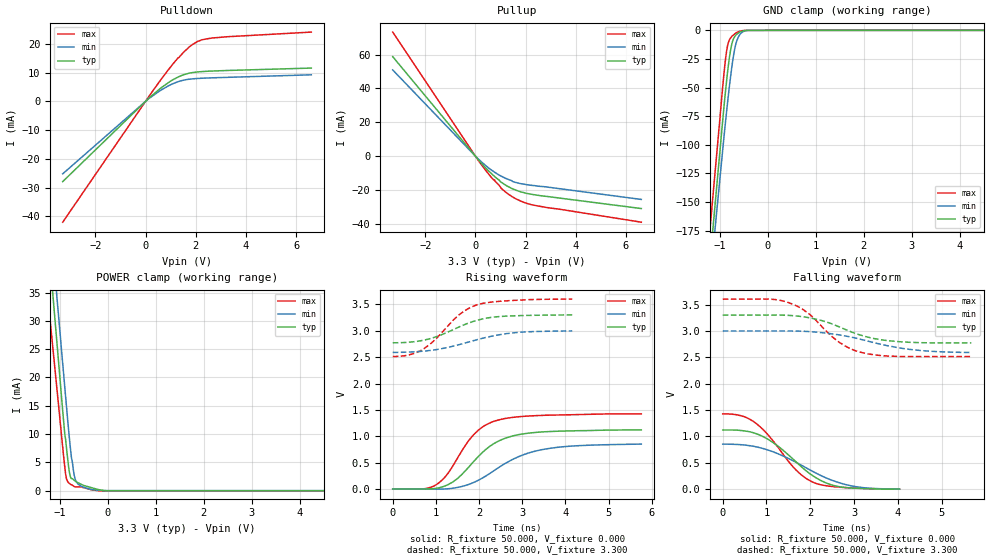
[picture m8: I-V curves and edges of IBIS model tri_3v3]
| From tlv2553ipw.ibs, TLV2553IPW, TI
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[Model]   tri_3v3
Model_type 3-state
Vref=0.000E+00
Rref=5.000E+06
Cref=3.000E-11
Vmeas=1.65E+00
C_comp  2.00000pF 2.00000pF 2.00000pF
[Voltage Range]   3.300E+00   3.000E+00   3.600E+00
[POWER Clamp Reference]   3.300E+00   3.000E+00   3.600E+00
[GND Clamp Reference]   0.000E+00   0.000E+00   0.000E+00
[Pullup Reference]   3.300E+00   3.000E+00   3.600E+00
[Pulldown Reference]   0.000E+00   0.000E+00   0.000E+00
[Temperature Range]   25   105   -40
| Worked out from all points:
|   slope of the pulldown table from 0 to 0.495 V, typ, clamps not added: 130 ohm
|   slope of the pullup table from 0 to 0.495 V, typ, clamps not added: 59.8 ohm
|   GND clamp passes 1 mA (typ) near -0.56 V on its own axis
|   POWER clamp passes 1 mA (typ) near -0.53 V on its own axis
|   rising waveform, R_fixture 50.000, V_fixture 0.000: 20-80 % time 888ps typ, 1.15ns min, 752ps max; typ from 0.001 V to 1.12 V
|   falling waveform, R_fixture 50.000, V_fixture 0.000: 20-80 % time 987ps typ, 1.26ns min, 867ps max; typ from 1.12 V to 0.001 V
|   rising waveform, R_fixture 50.000, V_fixture 3.300: 20-80 % time 969ps typ, 1.21ns min, 839ps max; typ from 2.77 V to 3.3 V
|   falling waveform, R_fixture 50.000, V_fixture 3.300: 20-80 % time 1.07ns typ, 1.37ns min, 895ps max; typ from 3.3 V to 2.77 V
[GND Clamp]
-3.3V     -1.173A    -1.124A    -1.155A
-1.02V    -115.5mA   -138.7mA   -86.59mA
-900mV    -60.5mA    -87.21mA   -31.75mA
-840mV    -36.62mA   -63.34mA   -13.37mA
-780mV    -17.99mA   -41.57mA   -6.751mA
-740mV    -10.19mA   -28.79mA   -4.811mA
-700mV    -6.094mA   -18.3mA    -3.44mA
-660mV    -3.764mA   -10.67mA   -2.16mA
-600mV    -1.942mA   -4.698mA   -1.006mA
-520mV    -523.6uA   -1.24mA    -186.4uA
-420mV    -6.897uA   -12.38uA   -383.5nA
6.6V      27.59uA    49.54uA    1.534uA
[Power Clamp]
-3.3V     249.5mA    251.4mA    209.7mA
-980mV    18.03mA    26.28mA    11mA
-900mV    10.16mA    18.46mA    4.361mA
-860mV    7.347mA    14.67mA    1.99mA
-820mV    4.34mA     10.89mA    1.379mA
-780mV    2.393mA    7.459mA    1.117mA
-760mV    2.109mA    5.878mA    1.021mA
-700mV    1.799mA    2.664mA    704.4uA
-660mV    1.562mA    1.592mA    648.6uA
-560mV    1.124mA    773.3uA    648.6uA
-80mV     13.44uA    115.4nA    -66.78uA
6.62V     -53.75uA   -461.7nA   -66.78uA
[Pullup]
-3.3V     58.78mA    50.94mA    73.31mA
80mV      -1.466mA   -1.235mA   -1.778mA
660mV     -10.64mA   -8.445mA   -12.97mA
720mV     -11.45mA   -9.069mA   -13.99mA
760mV     -11.98mA   -9.473mA   -13.99mA
980mV     -14.91mA   -11.48mA   -17.82mA
1.02V     -15.35mA   -11.77mA   -18.94mA
1.22V     -17.29mA   -13.22mA   -21.49mA
1.6V      -20.05mA   -15.54mA   -25.12mA
1.88V     -21.38mA   -16.42mA   -27.04mA
2.26V     -22.6mA    -17.31mA   -28.79mA
6.62V     -31mA      -25.61mA   -39.06mA
[Pulldown]
-3.3V     -27.89mA   -25.19mA   -41.99mA
140mV     1.176mA    1.05mA     1.784mA
620mV     4.685mA    3.925mA    7.645mA
1V        7.019mA    5.771mA    12mA
1.3V      8.455mA    6.827mA    15.16mA
1.74V     9.773mA    7.681mA    18.89mA
2.1V      10.23mA    7.953mA    20.94mA
2.66V     10.52mA    8.163mA    22mA
6.6V      11.55mA    9.212mA    24.05mA
[Rising Waveform]
R_fixture = 50.000
V_fixture = 0.000
V_fixture_min = 0.000
V_fixture_max = 0.000
|  time   V(typ)   V(min)   V(max)
0s        924.6uV    -1.577mV   1.993mV
720ps     209.3uV    -1.577mV   5.177mV
1.04ns    18.6mV     -1.826mV   99.87mV
1.24ns    68.18mV    3.409mV    254.6mV
1.48ns    186.8mV    27.05mV    558.2mV
1.88ns    526.5mV    126.1mV    1.035V
2.4ns     887.5mV    378.4mV    1.298V
2.96ns    1.038V     628.9mV    1.374V
3.52ns    1.086V     756.1mV    1.399V
5.76ns    1.121V     852.2mV    1.426V
[Falling Waveform]
R_fixture = 50.000
V_fixture = 0.000
V_fixture_min = 0.000
V_fixture_max = 0.000
|  time   V(typ)   V(min)   V(max)
0s        1.121V     852.2mV    1.426V
440ps     1.109V     840.1mV    1.386V
760ps     1.052V     802.2mV    1.248V
1.2ns     853.4mV    690.9mV    861.8mV
1.68ns    512.8mV    505.6mV    358.1mV
2.08ns    241mV      325.4mV    124mV
2.4ns     104.6mV    198.4mV    58.96mV
2.72ns    37.8mV     106mV      32.82mV
3.24ns    9.269mV    24.62mV    11.92mV
4.04ns    924.6uV    -1.577mV   1.993mV
[Rising Waveform]
R_fixture = 50.000
V_fixture = 3.300
V_fixture_min = 3.000
V_fixture_max = 3.600
|  time   V(typ)   V(min)   V(max)
0s        2.773V     2.59V      2.513V
360ps     2.783V     2.597V     2.54V
720ps     2.823V     2.615V     2.66V
960ps     2.875V     2.638V     2.815V
1.52ns    3.067V     2.734V     3.291V
1.76ns    3.148V     2.788V     3.425V
1.96ns    3.2V       2.833V     3.495V
2.28ns    3.255V     2.896V     3.544V
2.88ns    3.286V     2.969V     3.579V
4.16ns    3.301V     2.999V     3.602V
[Falling Waveform]
R_fixture = 50.000
V_fixture = 3.300
V_fixture_min = 3.000
V_fixture_max = 3.600
|  time   V(typ)   V(min)   V(max)
0s        3.301V     2.999V     3.602V
1.08ns    3.301V     2.999V     3.603V
1.56ns    3.292V     2.999V     3.52V
1.96ns    3.252V     2.988V     3.331V
2.68ns    3.069V     2.922V     2.774V
2.96ns    2.974V     2.878V     2.648V
3.24ns    2.898V     2.823V     2.577V
3.76ns    2.816V     2.72V      2.524V
4.36ns    2.782V     2.641V     2.513V
5.68ns    2.773V     2.59V      2.513V
[Ramp]
| variable typ min max
dV/dt_r 671.938m/936.235p 516.587m/1.23520n 854.418m/782.483p
dV/dt_f 315.804m/1.06255n 418.115m/1.35867n 654.459m/877.500p
R_load = 50.0000Ohms
